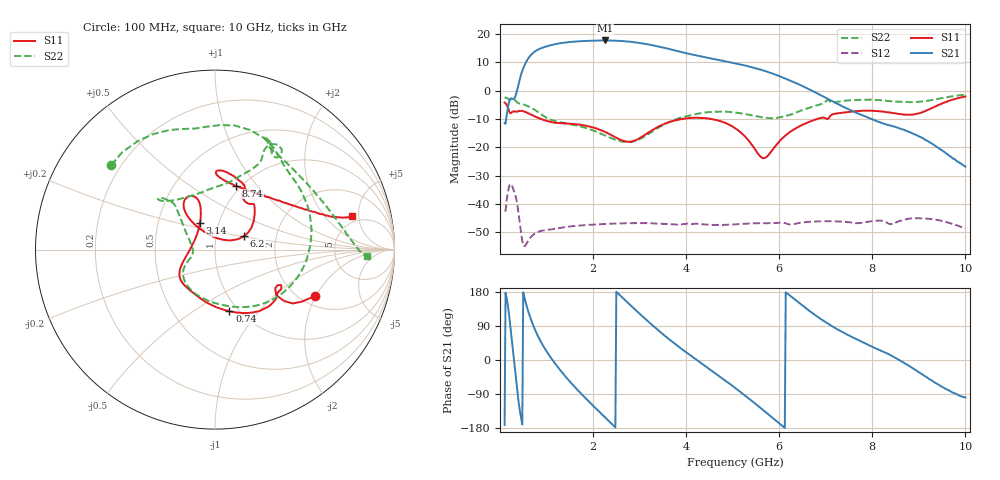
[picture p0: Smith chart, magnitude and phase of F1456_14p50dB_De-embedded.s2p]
! Integrated Device Technology
! Corporate Headquarters
! 6024 Silver Creek Valley Road
! San Jose, CA 95138  USA
! Phone:  1-408-284-8200
! Toll Free:  1-800-223-1366
! Webpage:  http://www.idt.com/
! Timing and RF Division
! 515 Groton Road, Suite 102
! Westford, MA 01886-6024
! Device:  F1456
! Description: 6-bit 0.5 dB Transmit Variable Gain Amplifier
! Frequency:  2100.0 -  2950.00 MHz
! Package:  6x6 mm Thin QFN Plastic Package: 28 pin
! State:  29
! Atten State:  14.5 dB
! Voltage:  +5.00 Volts
! Current:  216.986 mA
! Data:  The device was measured on a the F1455 evaluation board which has
!  individual transmission lines to the RF pins.  Data was collected
!  using a calibrated network analyzer.  The evaluation board was
!  de-embedded using a TRL calibration technique.
!  The reference plane is the edge of the package pin.
!  Pin  1 = CSb
!  Pin  2 = DATA
!  Pin  3 = CLK
!  Pin  4 = RSET
!  Pin  5 = GND
!  Pin  6 = RFIN  = Port 1
!  Pin  7 = GND
!  Pin  8 = NC
!  Pin  9 = NC
!  Pin 10 = NC
!  Pin 11 = NC
!  Pin 12 = NC
!  Pin 13 = NC
!  Pin 14 = /STBY
!  Pin 15 = GND
!  Pin 16 = RFOUT  = Port 2
!  Pin 17 = GND
!  Pin 18 = NC
!  Pin 19 = NC
!  Pin 20 = NC
!  Pin 21 = GND
!  Pin 22 = NC
!  Pin 23 = GND
!  Pin 24 = NC
!  Pin 25 = NC
!  Pin 26 = NC
!  Pin 27 = GND
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# GHz S dB R 50
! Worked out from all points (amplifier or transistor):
!   496 points, 100 MHz to 10 GHz, reference 50 ohm
!   highest |S21| = 17.6 dB at 2.26 GHz (marker M1)
!   |S21| within 3 dB of that: 846 MHz to 3.633 GHz (2.787 GHz wide, 124 % of centre)
!   unconditionally stable (mu >= 1): start of sweep to end of sweep
!   at 1.74 GHz: K = 14.35, MAG = 17.9 dB, |S12| = -47.5 dB
!   at 5.06 GHz: K = 30.08, MAG = 10.6 dB, |S12| = -47.1 dB
!   at 10 GHz: K = 321.14, MAG = -17.2 dB, |S12| = -48.5 dB
!   S11 on the Smith chart (normalised r, x): 100 MHz: 2.36, -1.97; 740 MHz: 0.91, -0.71; 3.14 GHz: 0.81, +0.25; 6.2 GHz: 1.37, +0.21; 8.74 GHz: 0.95, +0.79; 10 GHz: 4.23, +4.07
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0.1  -4.23 -25.0  -11.43 -171.7  -42.34 47.6  -2.56 140.9
0.32  -7.38 -32.2  -2.51 -21.3  -36.34 -146.4  -3.35 66.5
0.44  -7.18 -41.8  4.83 -143.4  -48.41 137.6  -4.66 38.5
0.58  -7.79 -59.1  10.57 139.8  -53.68 164.3  -5.37 6.7
0.74  -9.06 -76.9  13.62 83.8  -50.47 135.9  -6.72 -27.7
0.96  -10.50 -98.5  15.34 30.9  -49.24 94.7  -9.20 -67.5
1.18  -11.34 -115.7  16.30 -8.6  -48.70 69.4  -10.76 -95.7
1.48  -11.67 -132.3  17.06 -53.8  -47.95 43.9  -11.78 -123.8
1.76  -12.14 -143.1  17.39 -90.9  -47.50 25.3  -12.78 -140.5
2.26  -14.60 -160.3  17.63 -151.7  -47.02 -2.3  -15.85 -157.6
2.64  -17.67 171.4  17.42 163.6  -46.79 -21.6  -18.05 -170.9
3.14  -15.32 119.2  16.38 106.5  -46.73 -46.7  -15.83 156.2
3.4  -12.74 110.1  15.53 78.5  -46.88 -58.9  -13.18 143.0
3.74  -10.63 108.9  14.21 44.4  -47.17 -73.5  -10.37 133.8
4.08  -9.69 113.9  12.84 13.3  -47.04 -88.5  -8.81 132.6
5.06  -13.33 129.7  9.57 -74.3  -47.14 -131.8  -7.76 138.0
5.66  -23.83 75.2  7.06 -132.8  -46.75 -165.1  -9.50 120.2
6.2  -14.96 25.1  3.70 173.0  -47.11 161.8  -8.69 81.8
6.7  -10.68 41.1  -0.04 125.0  -46.21 137.2  -5.77 64.1
8.36  -7.71 87.9  -12.20 14.9  -46.96 66.5  -3.76 62.4
8.74  -8.52 71.8  -14.25 -12.1  -45.29 59.5  -4.08 49.1
10  -2.11 13.7  -26.81 -98.7  -48.50 -24.1  -1.46 -2.6
